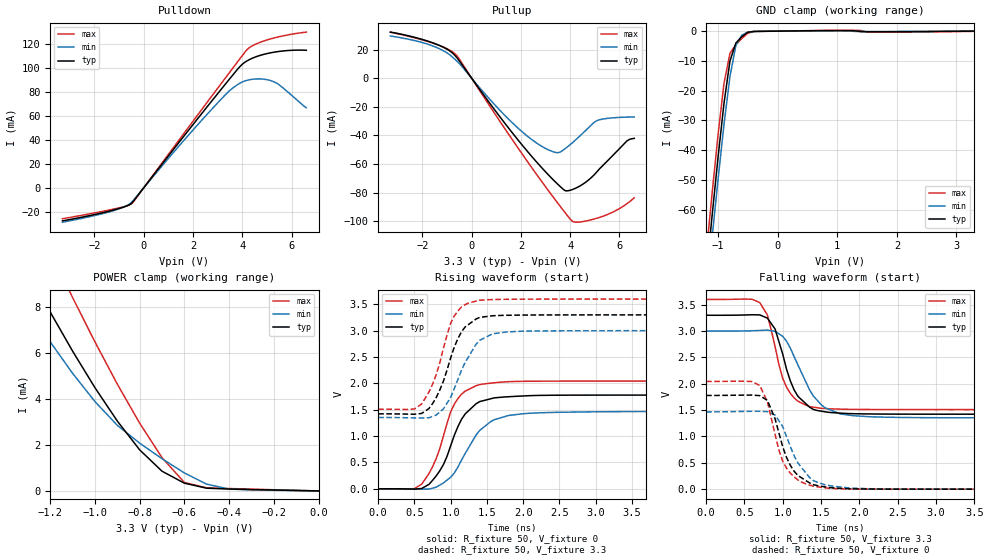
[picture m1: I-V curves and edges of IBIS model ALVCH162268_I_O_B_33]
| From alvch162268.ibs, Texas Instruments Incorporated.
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|************* ALVCH162268 OUTPUT (3.3 V) MODEL**************
[Model]   ALVCH162268_I_O_B_33
Model_type  I/O
Polarity   Non-Inverting
Enable   Active-Low
Vinl = 0.8V
Vinh = 2.0V
Vmeas = 1.5V
Cref = 50pF
Rref = 500
Vref = 0
| variable   typ   min   max
C_comp   8.15pF   NA   NA
[Temperature Range]   50   100   0
[Voltage range]   3.3   3   3.6
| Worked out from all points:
|   slope of the pulldown table from 0 to 0.495 V, typ, clamps not added: 37.4 ohm
|   slope of the pullup table from 0 to 0.495 V, typ, clamps not added: 41.7 ohm
|   GND clamp passes 1 mA (typ) near -0.54 V on its own axis
|   POWER clamp passes 1 mA (typ) near -0.72 V on its own axis
|   rising waveform, R_fixture 50, V_fixture 0: 20-80 % time 345ps typ, 414ps min, 317ps max; typ from 0 V to 1.78 V
|   falling waveform, R_fixture 50, V_fixture 3.3: 20-80 % time 260ps typ, 351ps min, 231ps max; typ from 3.3 V to 1.42 V
|   rising waveform, R_fixture 50, V_fixture 3.3: 20-80 % time 305ps typ, 343ps min, 284ps max; typ from 1.42 V to 3.3 V
|   falling waveform, R_fixture 50, V_fixture 0: 20-80 % time 267ps typ, 306ps min, 242ps max; typ from 1.78 V to 0 V
|Process range|   weak   strong
[Pullup]
|   50C:3.3V:   100C:3V:weak   0C:3.6V:strong
|   Voltage   I(typ)   I(min)   I(max)
-3.3V     32.3mA     29.56mA    32.19mA
-1.6V     24.88mA    22.74mA    24.76mA
-1V       20.31mA    17.76mA    20.61mA
-600mV    14.41mA    11.97mA    15.84mA
1.1V      -25.91mA   -21.57mA   -28.91mA
2.3V      -51.88mA   -41.02mA   -59.12mA
3.3V      -70.84mA   -51.37mA   -82.9mA
3.8V      -78.7mA    -49.18mA   -94.18mA
4.2V      -77.06mA   -43.4mA    -100.6mA
5.1V      -65.09mA   -29.56mA   -97.81mA
6.3V      -43.88mA   -27.17mA   -87.76mA
6.6V      -42.02mA   -27.06mA   -83.57mA
[Pulldown]
|   50C:3.3V:   100C:3V:weak   0C:3.6V:strong
|   Voltage   I(typ)   I(min)   I(max)
-3.3V     -27.73mA   -28.82mA   -25.9mA
-1.3V     -19.05mA   -19.58mA   -18.16mA
-800mV    -16.01mA   -16.04mA   -15.93mA
-500mV    -13.15mA   -12.26mA   -13.47mA
2.7V      71.04mA    64.38mA    75.01mA
3.5V      91.47mA    81.57mA    96.95mA
4V        103.3mA    88.51mA    110.6mA
4.2V      106.3mA    89.93mA    115.8mA
4.4V      108.3mA    90.76mA    118.7mA
4.9V      111.8mA    90.78mA    123mA
5.3V      113.5mA    88.51mA    125.4mA
6.6V      115mA      66.9mA     130.3mA
[GND Clamp]
|   50C:3.3V:   100C:3V:weak   0C:3.6V:strong
|   Voltage   I(typ)   I(min)   I(max)
-3.3V     -542mA     -543.9mA   -539.4mA
-1.2V     -82.62mA   -89.68mA   -75.36mA
-1.1V     -62.18mA   -69.47mA   -54.67mA
-1V       -42.47mA   -49.89mA   -34.92mA
-900mV    -24.28mA   -31.41mA   -17.54mA
-800mV    -10.02mA   -15.26mA   -7.48mA
-700mV    -3.978mA   -4.726mA   -4.539mA
-600mV    -1.856mA   -1.312mA   -2.446mA
-500mV    -377.3uA   -311.4uA   -707.6uA
-400mV    -109.7uA   -99.23uA   -141.6uA
900mV     182.4uA    116.3uA    254.7uA
3.3V      159.2pA    44.74uA    -73.47uA
[POWER Clamp]
|   50C:3.3V:   100C:3V:weak   0C:3.6V:strong
|   Voltage   I(typ)   I(min)   I(max)
-3.3V     52.65mA    46.37mA    59.41mA
-1.4V     11.43mA    9.537mA    14.61mA
-1.3V     9.573mA    7.971mA    12.49mA
-1.2V     7.789mA    6.492mA    10.43mA
-1.1V     6.089mA    5.122mA    8.423mA
-900mV    3.043mA    2.856mA    4.652mA
-800mV    1.788mA    2.081mA    2.95mA
-700mV    858.2uA    1.403mA    1.447mA
-600mV    337.7uA    782.8uA    367.8uA
-500mV    119.1uA    293.9uA    133.6uA
-400mV    82.07uA    81.73uA    103.7uA
0V        154.3pA    691.3pA    84.99pA
[ramp]
| variable   typ   min   max
dV/dt_r   1.0701E+00/3.4572E-10  8.8383E-01/4.1539E-10  1.2286E+00/3.1570E-10
dV/dt_f   1.1318E+00/2.5060E-10  9.9922E-01/3.5321E-10  1.2580E+00/2.3133E-10
[Rising Waveform]
R_fixture = 50
V_fixture = 0
V_fixture_min = 0
V_fixture_max = 0
C_fixture = 0
L_fixture = 0
|   50C:3.3V:   100C:3V:weak   0C:3.6V:strong
|   Time   V(typ)   V(min)   V(max)
0s        0V         0V         0V
500ps     -5.169mV   -2.871mV   4.379mV
700ps     84.57mV    -4.717mV   288.6mV
900ps     460.7mV    111.7mV    1.005V
1ns       818.5mV    220.8mV    1.463V
1.1ns     1.182V     413.4mV    1.714V
1.35ns    1.614V     1.022V     1.956V
1.6ns     1.726V     1.311V     2.013V
3.1ns     1.778V     1.462V     2.044V
13.5ns    1.778V     1.467V     2.044V
[Falling Waveform]
R_fixture = 50
V_fixture = 3.3
V_fixture_min = 3
V_fixture_max = 3.6
C_fixture = 0
L_fixture = 0
|   50C:3.3V:   100C:3V:weak   0C:3.6V:strong
|   Time   V(typ)   V(min)   V(max)
0s        3.3V       3V         3.6V
600ps     3.308V     3.005V     3.603V
800ps     3.244V     3.018V     3.303V
900ps     3.037V     2.994V     2.705V
1.05ns    2.272V     2.806V     1.933V
1.2ns     1.758V     2.35V      1.667V
1.5ns     1.48V      1.605V     1.534V
1.8ns     1.438V     1.417V     1.516V
2.6ns     1.423V     1.359V     1.51V
13.5ns    1.422V     1.353V     1.51V
[Rising Waveform]
R_fixture = 50
V_fixture = 3.3
V_fixture_min = 3
V_fixture_max = 3.6
C_fixture = 0
L_fixture = 0
|   50C:3.3V:   100C:3V:weak   0C:3.6V:strong
|   Time   V(typ)   V(min)   V(max)
0s        1.422V     1.353V     1.51V
500ps     1.415V     1.345V     1.515V
700ps     1.523V     1.348V     1.837V
800ps     1.73V      1.399V     2.165V
900ps     2.044V     1.516V     2.669V
1.05ns    2.691V     1.904V     3.28V
1.2ns     3.072V     2.4V       3.495V
1.4ns     3.252V     2.817V     3.578V
2.25ns    3.298V     2.995V     3.599V
13.5ns    3.3V       3V         3.6V
[Falling Waveform]
R_fixture = 50
V_fixture = 0
V_fixture_min = 0
V_fixture_max = 0
C_fixture = 0
L_fixture = 0
|   50C:3.3V:   100C:3V:weak   0C:3.6V:strong
|   Time   V(typ)   V(min)   V(max)
0s        1.778V     1.467V     2.044V
600ps     1.785V     1.477V     2.041V
700ps     1.774V     1.478V     1.966V
800ps     1.684V     1.47V      1.658V
950ps     1.065V     1.296V     741.8mV
1.05ns    599mV      994.8mV    397.2mV
1.2ns     256.6mV    492.7mV    173mV
1.35ns    118mV      219.9mV    76.3mV
1.6ns     32.11mV    70.71mV    17.2mV
13.5ns    3.278uV    3.476uV    2.132uV
